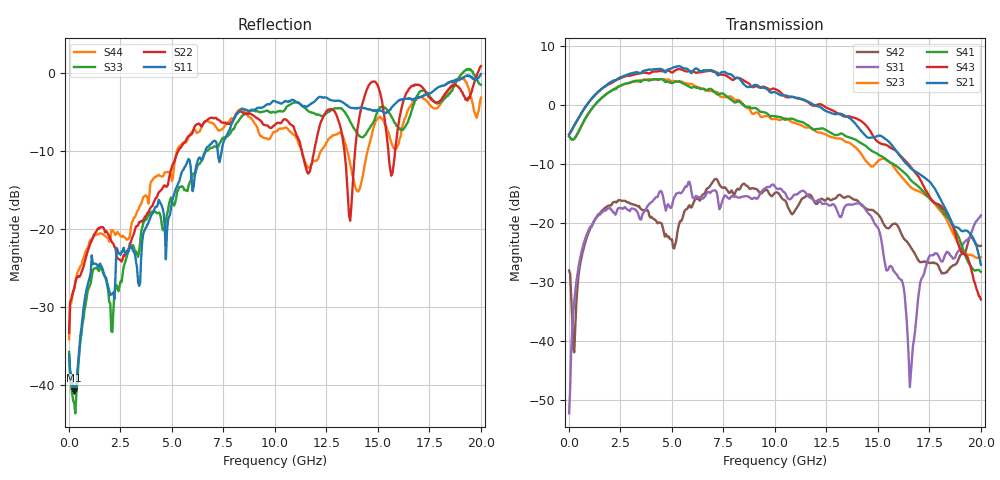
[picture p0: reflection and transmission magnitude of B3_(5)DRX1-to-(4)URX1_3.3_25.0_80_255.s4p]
!Agilent Technologies,N5225A,MY51451112,A.09.50.13
!Agilent N5225A: A.09.50.13
!Date: Sunday, March 12, 2017 05:23:25
!Correction: S11(Full 4 Port(1,2,3,4))
!S12(Full 4 Port(1,2,3,4))
!S13(Full 4 Port(1,2,3,4))
!S14(Full 4 Port(1,2,3,4))
!S21(Full 4 Port(1,2,3,4))
!S22(Full 4 Port(1,2,3,4))
!S23(Full 4 Port(1,2,3,4))
!S24(Full 4 Port(1,2,3,4))
!S31(Full 4 Port(1,2,3,4))
!S32(Full 4 Port(1,2,3,4))
!S33(Full 4 Port(1,2,3,4))
!S34(Full 4 Port(1,2,3,4))
!S41(Full 4 Port(1,2,3,4))
!S42(Full 4 Port(1,2,3,4))
!S43(Full 4 Port(1,2,3,4))
!S44(Full 4 Port(1,2,3,4))
!S4P File: Measurements: <S11,S12,S13,S14>,
!<S21,S22,S23,S24>,
!<S31,S32,S33,S34>,
!<S41,S42,S43,S44>:
# Hz S  dB  R 50
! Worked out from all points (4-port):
!   401 points, 10 MHz to 20 GHz, reference 50 ohm
!   strongest paths, dB at 10 MHz, 5.008 GHz, 10.01 GHz, 15 GHz, 20 GHz:
!     S21: -5.0, 6.2, 2.1, -5.2, -27.1
!     S43: -5.0, 5.4, 2.7, -6.3, -33.0
!     S41: -5.3, 3.6, -1.9, -8.4, -28.3
!     S23: -5.3, 4.0, -2.4, -9.5, -25.8
!     S31: -52.2, -17.1, -13.8, -20.8, -18.7
!     S42: -28.0, -22.8, -14.9, -18.5, -23.9
!   lowest |S11| = -40.7 dB at 259.9 MHz (marker M1), VSWR 1.02, Z = 50.3 - j0.879 ohm
!   |S11| at or under -10 dB: start of sweep to 6.625 GHz; 7.221 GHz to 7.416 GHz (195.1 MHz wide, 2.67 % of centre)
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1e7  -36.11 -38.9  -62.77 108.5  -53.81 19.5  -66.33 132.7
     -5.01 2.1  -33.31 39.2  -5.33 -179.3  -28.00 38.0
     -52.22 20.2  -69.43 159.6  -35.74 -47.1  -69.76 106.3
     -5.33 -179.3  -28.05 38.1  -4.99 2.2  -34.11 44.9
2.59875e8  -40.71 -71.5  -49.87 56.0  -33.09 94.9  -50.59 54.5
           -3.50 8.1  -27.61 -132.0  -5.75 -176.5  -41.75 -162.4
           -33.20 95.5  -49.84 56.8  -42.30 -78.5  -50.55 55.1
           -5.75 -177.3  -41.91 -170.7  -3.48 7.4  -27.62 -138.0
2.858575e9  -22.84 149.8  -39.08 -36.0  -17.68 54.7  -37.94 -46.4
            5.14 -90.8  -22.79 157.5  3.66 82.5  -16.34 42.2
            -17.78 54.4  -38.53 -29.0  -23.09 126.1  -37.55 -37.7
            3.67 72.7  -16.51 41.5  4.92 -98.8  -21.27 138.6
4.957525e9  -17.34 96.3  -42.34 -32.3  -16.80 29.5  -37.76 -19.6
            6.14 171.0  -12.40 149.9  4.02 -24.7  -24.48 28.4
            -17.47 21.3  -40.10 3.3  -15.97 108.2  -35.01 6.5
            3.68 -40.3  -22.78 39.2  5.54 158.0  -13.04 116.0
7.956025e9  -6.25 41.3  -32.69 -102.0  -16.56 8.3  -31.96 -122.0
            4.90 21.1  -6.15 88.6  1.18 -166.5  -14.39 50.6
            -15.53 6.6  -29.95 -102.3  -7.22 64.8  -30.65 -132.8
            0.66 168.4  -14.90 48.0  4.19 9.9  -5.96 42.9
1.155422e10  -4.34 -6.0  -37.42 -117.6  -14.65 -22.4  -40.05 -136.9
             0.63 -134.5  -12.61 85.2  -3.83 39.4  -15.39 37.0
             -15.20 -23.5  -33.54 -123.2  -4.75 10.5  -34.10 -152.1
             -3.39 1.7  -15.35 42.7  0.56 -159.4  -11.86 25.4
2e10  -0.17 -114.2  -32.94 62.9  -18.76 121.3  -35.46 21.8
      -27.07 -164.9  0.84 17.1  -25.79 20.2  -23.89 102.0
      -18.72 121.2  -34.00 40.4  -1.53 -87.7  -35.24 -7.7
      -28.27 -28.8  -23.87 102.9  -32.95 163.2  -3.18 -136.7
